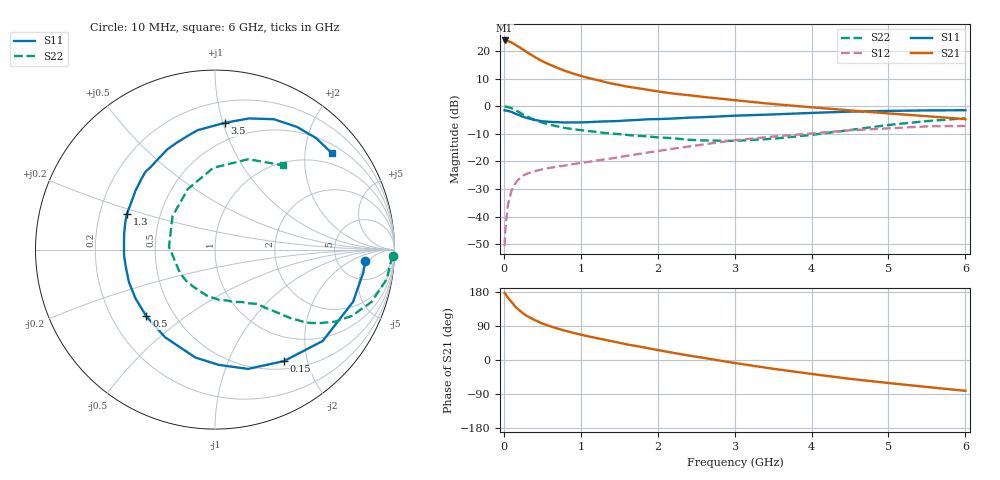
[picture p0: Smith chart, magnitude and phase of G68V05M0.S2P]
! SIEMENS Small Signal Semiconductors
! BFG193
! Si NPN RF Bipolar Junction Transistor in SOT223
! VCE = 8 V  IC = 5 mA
! Common Emitter S-Parameters:  August  1996
# GHz  S  MA  R  50
!  f  S11  S21  S12  S22
! GHz  MAG  ANG  MAG  ANG  MAG  ANG  MAG  ANG
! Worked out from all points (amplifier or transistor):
!   36 points, 10 MHz to 6 GHz, reference 50 ohm
!   highest |S21| = 23.8 dB at 10 MHz (marker M1)
!   |S21| within 3 dB of that: start of sweep to 232.8 MHz
!   unconditionally stable (mu >= 1): 1.137 GHz to 2.543 GHz
!   at 250 MHz: K = 0.34, MSG = 22.9 dB, |S12| = -25.2 dB
!   at 1.4 GHz: K = 1.08, MAG = 11.8 dB, |S12| = -19.0 dB
!   at 6 GHz: K = 0.86, MSG = 1.2 dB, |S12| = -7.2 dB
!   S11 on the Smith chart (normalised r, x): 10 MHz: 10, -4; 150 MHz: 0.61, -1.62; 500 MHz: 0.35, -0.36; 1.3 GHz: 0.32, +0.17; 3.5 GHz: 0.36, +1.01; 6 GHz: 0.70, +2.63
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0.01  0.8401 -4.2  15.54 176.8  0.0029 91.3  0.991 -2.0
0.02  0.8361 -8.8  15.53 174.7  0.0059 86.4  0.9822 -4.0
0.05  0.8225 -20.7  15.22 165.0  0.0155 78.1  0.9708 -9.8
0.1  0.7871 -40.3  14.29 153.2  0.0294 69.8  0.9193 -18.5
0.15  0.7303 -58.3  12.99 140.5  0.0402 61.4  0.8466 -25.9
0.2  0.6898 -74.5  11.79 131.6  0.0485 55.8  0.7796 -31.0
0.25  0.6428 -88.1  10.61 123.0  0.055 50.5  0.7083 -35.4
0.3  0.6113 -100.3  9.547 116.2  0.0595 47.6  0.6546 -38.5
0.4  0.5622 -119.6  7.82 105.6  0.0659 43.0  0.5639 -42.4
0.5  0.5337 -135.8  6.523 96.3  0.0717 40.0  0.5028 -44.9
0.6  0.5193 -148.6  5.643 89.2  0.0763 39.6  0.4611 -47.0
0.7  0.5128 -159.2  4.935 82.8  0.0802 38.9  0.4292 -49.1
0.9  0.5078 -176.2  3.905 71.8  0.0892 38.8  0.3833 -52.3
1.1  0.5141 169.9  3.248 62.4  0.0979 39.8  0.3546 -57.6
1.3  0.5299 158.1  2.78 53.9  0.1083 40.0  0.3288 -62.6
1.6  0.5514 143.4  2.271 41.1  0.1259 39.3  0.302 -72.9
2.2  0.5977 121.5  1.694 19.0  0.1693 34.7  0.2634 -98.7
2.8  0.6518 103.4  1.377 -1.3  0.222 26.1  0.2367 -133.5
3.5  0.7085 85.6  1.093 -23.1  0.2818 11.5  0.257 176.4
4.5  0.7971 65.7  0.839 -49.7  0.3658 -9.0  0.3697 114.2
5.5  0.8385 47.9  0.658 -71.2  0.4305 -35.3  0.5369 69.7
6  0.8443 39.4  0.583 -81.3  0.4384 -50.2  0.6045 50.9
